(* Logix 5000 DataType export AMCI_NXEE2_Output_Data; software revision 20.05 *)

TYPE AMCI_NXEE2_Output_Data :
STRUCT
   Command_Word : INT;
   Configuration_Word : INT;
   Number_of_SSI_Data_Bits : INT;
   Number_Of_Data_Value_Bits : SINT;
   MSB_Number : SINT;
   Scalar_Multiplier : INT;
   Scalar_Divisor : INT;
   Preset_Value : DINT;
   Full_Scale_Count : DINT;
END_STRUCT
END_TYPE
